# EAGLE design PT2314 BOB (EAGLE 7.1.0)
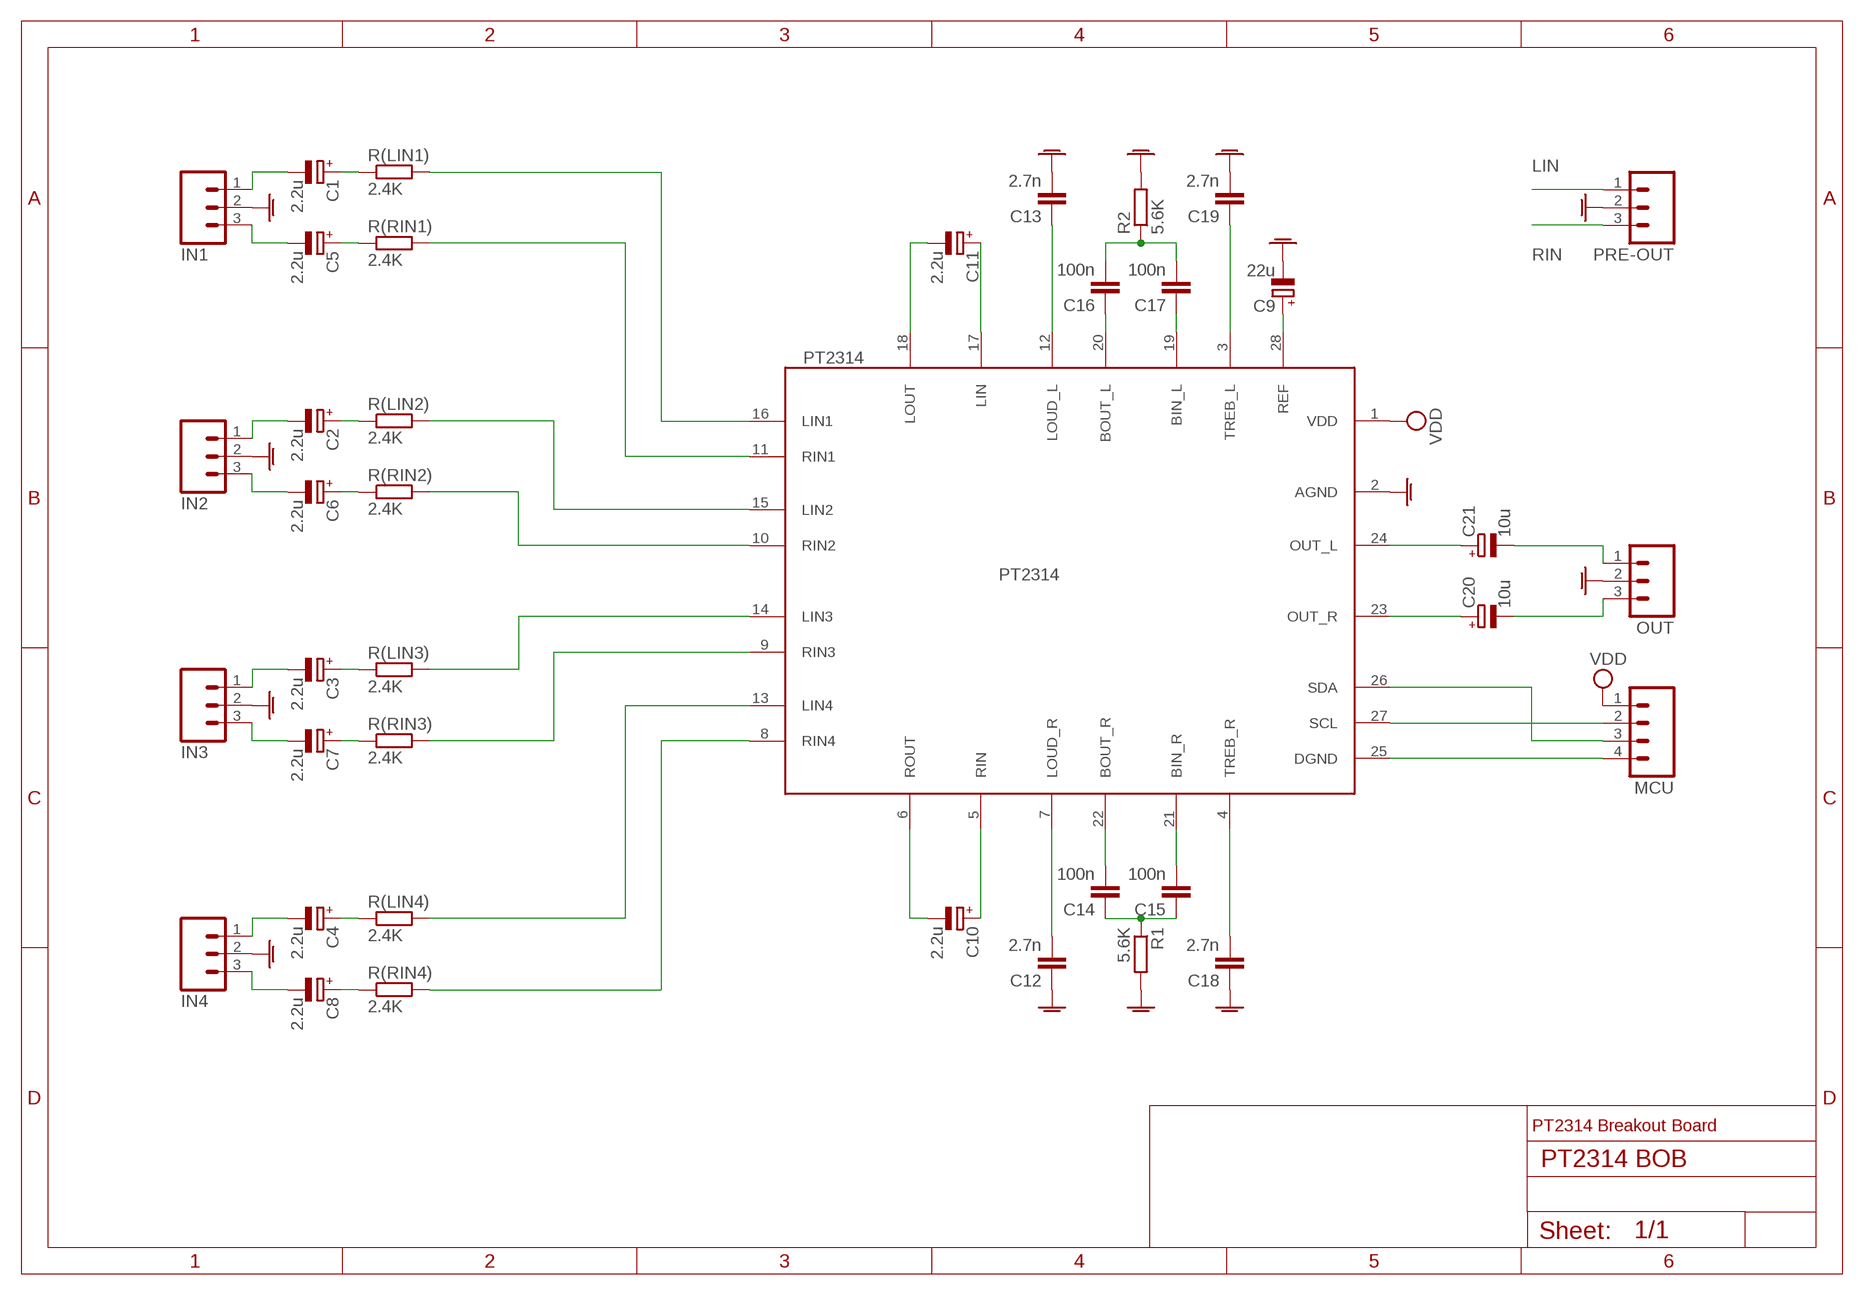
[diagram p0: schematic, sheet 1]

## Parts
C1  2.2u  CPOL-EUSMCZ  [SMC_Z]
C2  2.2u  CPOL-EUSMCZ  [SMC_Z]
C3  2.2u  CPOL-EUSMCZ  [SMC_Z]
C4  2.2u  CPOL-EUSMCZ  [SMC_Z]
C5  2.2u  CPOL-EUSMCZ  [SMC_Z]
C6  2.2u  CPOL-EUSMCZ  [SMC_Z]
C7  2.2u  CPOL-EUSMCZ  [SMC_Z]
C8  2.2u  CPOL-EUSMCZ  [SMC_Z]
C9  22u  CPOL-EUSMCZ  [SMC_Z]
C10  2.2u  CPOL-EUSMCZ  [SMC_Z]
C11  2.2u  CPOL-EUSMCZ  [SMC_Z]
C12  2.7n  C-EUC0603  [C0603]
C13  2.7n  C-EUC0603  [C0603]
C14  100n  C-EUC0603  [C0603]
C15  100n  C-EUC0603  [C0603]
C16  100n  C-EUC0603  [C0603]
C17  100n  C-EUC0603  [C0603]
C18  2.7n  C-EUC0603  [C0603]
C19  2.7n  C-EUC0603  [C0603]
C20  10u  CPOL-EUSMCZ  [SMC_Z]
C21  10u  CPOL-EUSMCZ  [SMC_Z]
IN1  M03PTH  [1X03]
IN2  M03PTH  [1X03]
IN3  M03PTH  [1X03]
IN4  M03PTH  [1X03]
MCU  M04PTH  [1X04]
OUT  M03PTH  [1X03]
PRE-OUT  M03PTH  [1X03]
PT2314  PT2314  [SO-28W]
R1  5.6K  R-EU_R0603  [R0603]
R2  5.6K  R-EU_R0603  [R0603]
R(LIN1)  2.4K  R-EU_R0603  [R0603]
R(LIN2)  2.4K  R-EU_R0603  [R0603]
R(LIN3)  2.4K  R-EU_R0603  [R0603]
R(LIN4)  2.4K  R-EU_R0603  [R0603]
R(RIN1)  2.4K  R-EU_R0603  [R0603]
R(RIN2)  2.4K  R-EU_R0603  [R0603]
R(RIN3)  2.4K  R-EU_R0603  [R0603]
R(RIN4)  2.4K  R-EU_R0603  [R0603]

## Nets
AGND: C9.- C12.1 C13.2 C18.1 C19.2 IN1.2 IN2.2 IN3.2 IN4.2 OUT.2 PRE-OUT.2 PT2314.2(AGND) R1.2 R2.2
B[IN|OUT]_L: C16.2 C17.2 R2.1
B[IN|OUT]_R: C14.1 C15.1 R1.1
BIN_L: C17.1 PT2314.19(BIN_L)
BIN_R: C15.2 PT2314.21(BIN_R)
BOUT_L: C16.1 PT2314.20(BOUT_L)
BOUT_R: C14.2 PT2314.22(BOUT_R)
C1-IN1_L: C1.- IN1.1
C1-R: C1.+ R(LIN1).1
C2-IN2_L: C2.- IN2.1
C2-R: C2.+ R(LIN2).1
C3-IN3_L: C3.- IN3.1
C3-R: C3.+ R(LIN3).1
C4-IN4_L: C4.- IN4.1
C4-R: C4.+ R(LIN4).1
C5-IN1_R: C5.- IN1.3
C5-R: C5.+ R(RIN1).1
C6-IN2_R: C6.- IN2.3
C6-R: C6.+ R(RIN2).1
C7-IN3_R: C7.- IN3.3
C7-R: C7.+ R(RIN3).1
C8-IN4_R: C8.- IN4.3
C8-R: C8.+ R(RIN4).1
C20-OUT_R: C20.- OUT.3
C21-OUT_L: C21.- OUT.1
DGND: MCU.4 PT2314.25(DGND)
LIN: C11.+ PRE-OUT.1 PT2314.17(LIN)
LIN1: PT2314.16(LIN1) R(LIN1).2
LIN2: PT2314.15(LIN2) R(LIN2).2
LIN3: PT2314.14(LIN3) R(LIN3).2
LIN4: PT2314.13(LIN4) R(LIN4).2
LOUT: C11.- PT2314.18(LOUT)
N$1: C19.1 PT2314.3(TREB_L)
N$2: C13.1 PT2314.12(LOUD_L)
N$3: C18.2 PT2314.4(TREB_R)
N$4: C12.2 PT2314.7(LOUD_R)
OUT_L: C21.+ PT2314.24(OUT_L)
OUT_R: C20.+ PT2314.23(OUT_R)
REF: C9.+ PT2314.28(REF)
RIN: C10.+ PRE-OUT.3 PT2314.5(RIN)
RIN1: PT2314.11(RIN1) R(RIN1).2
RIN2: PT2314.10(RIN2) R(RIN2).2
RIN3: PT2314.9(RIN3) R(RIN3).2
RIN4: PT2314.8(RIN4) R(RIN4).2
ROUT: C10.- PT2314.6(ROUT)
SCL: MCU.2 PT2314.27(SCL)
SDA: MCU.3 PT2314.26(SDA)
VDD: MCU.1 PT2314.1(VDD)

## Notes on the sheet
- PT2314 Breakout Board

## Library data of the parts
C1-C11 C20 C21 = rcl:CPOL-EU: POLARIZED CAPACITOR, European symbol
C12-C19 = rcl:C-EU: CAPACITOR, European symbol
IN1-IN4 OUT PRE-OUT = SparkFun-Connectors:M03: Header 3 Standard 3-pin 0.1" header. Use with straight break away headers (SKU : PRT-00116), right angle break away headers (PRT-00553), swiss pins (PRT-00743), machine pins (PRT-00117), and female headers (PRT-00115). Molex polarized connector foot print use with SKU : PRT-08232 with associated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
MCU = SparkFun-Connectors:M04: Header 4 Standard 4-pin 0.1" header. Use with straight break away headers (SKU : PRT-00116), right angle break away headers (PRT-00553), swiss pins (PRT-00743), machine pins (PRT-00117), and female headers (PRT-00115). Molex polarized connector foot print use with SKU : PRT-08231 with associated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
PT2314 = audio-mixer-processor:PT2314: 4-Channel Input Audio Processor
R1 R2 R(LIN1) R(LIN2) R(LIN3) R(LIN4) R(RIN1) R(RIN2) R(RIN3) R(RIN4) = rcl:R-EU_: RESISTOR, European symbol

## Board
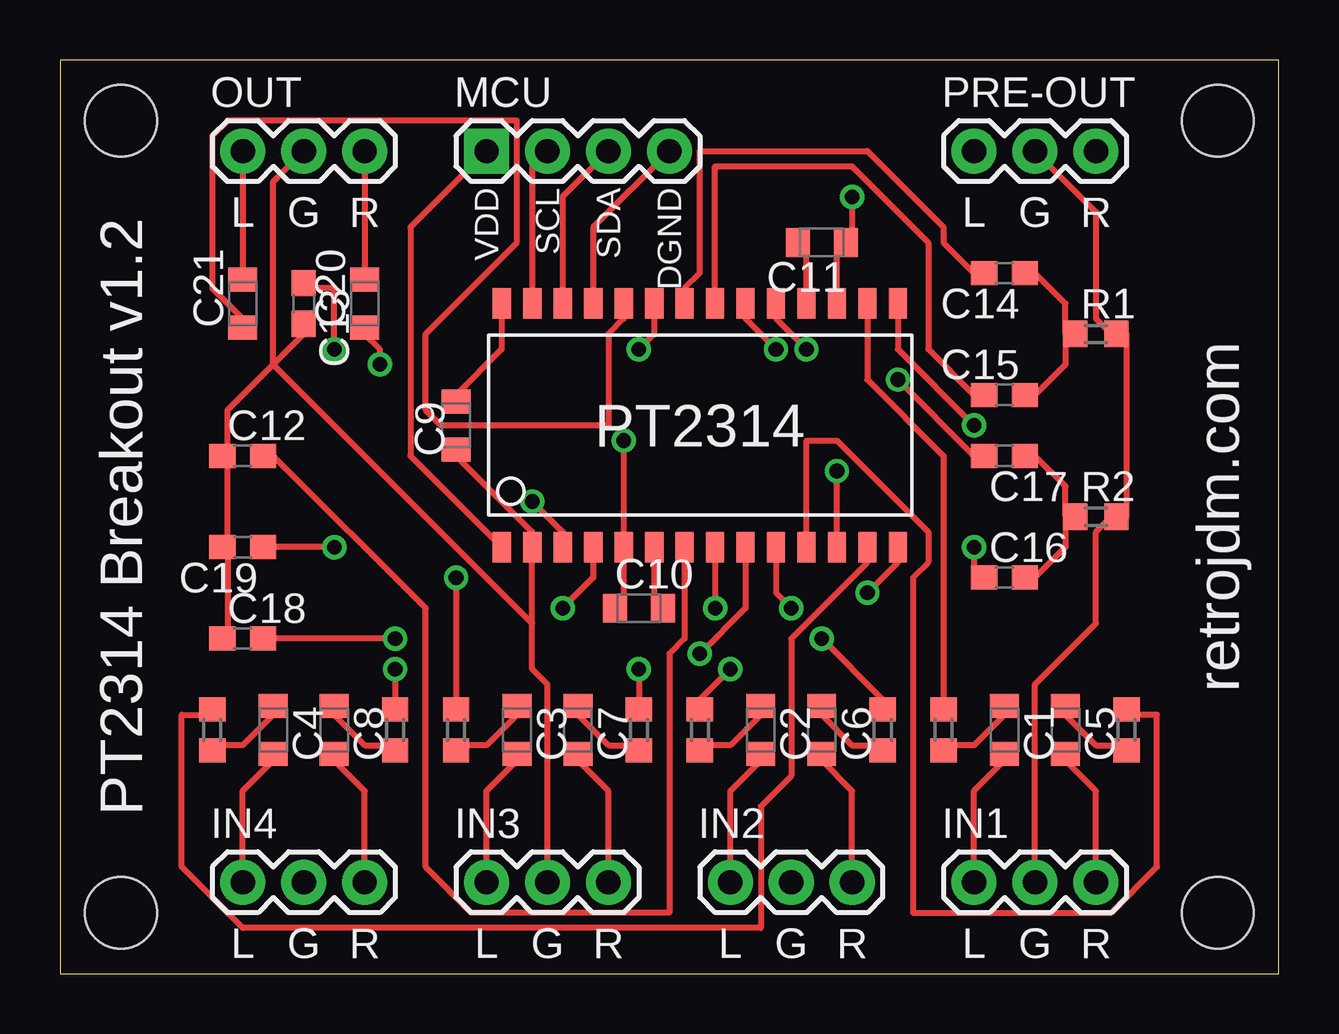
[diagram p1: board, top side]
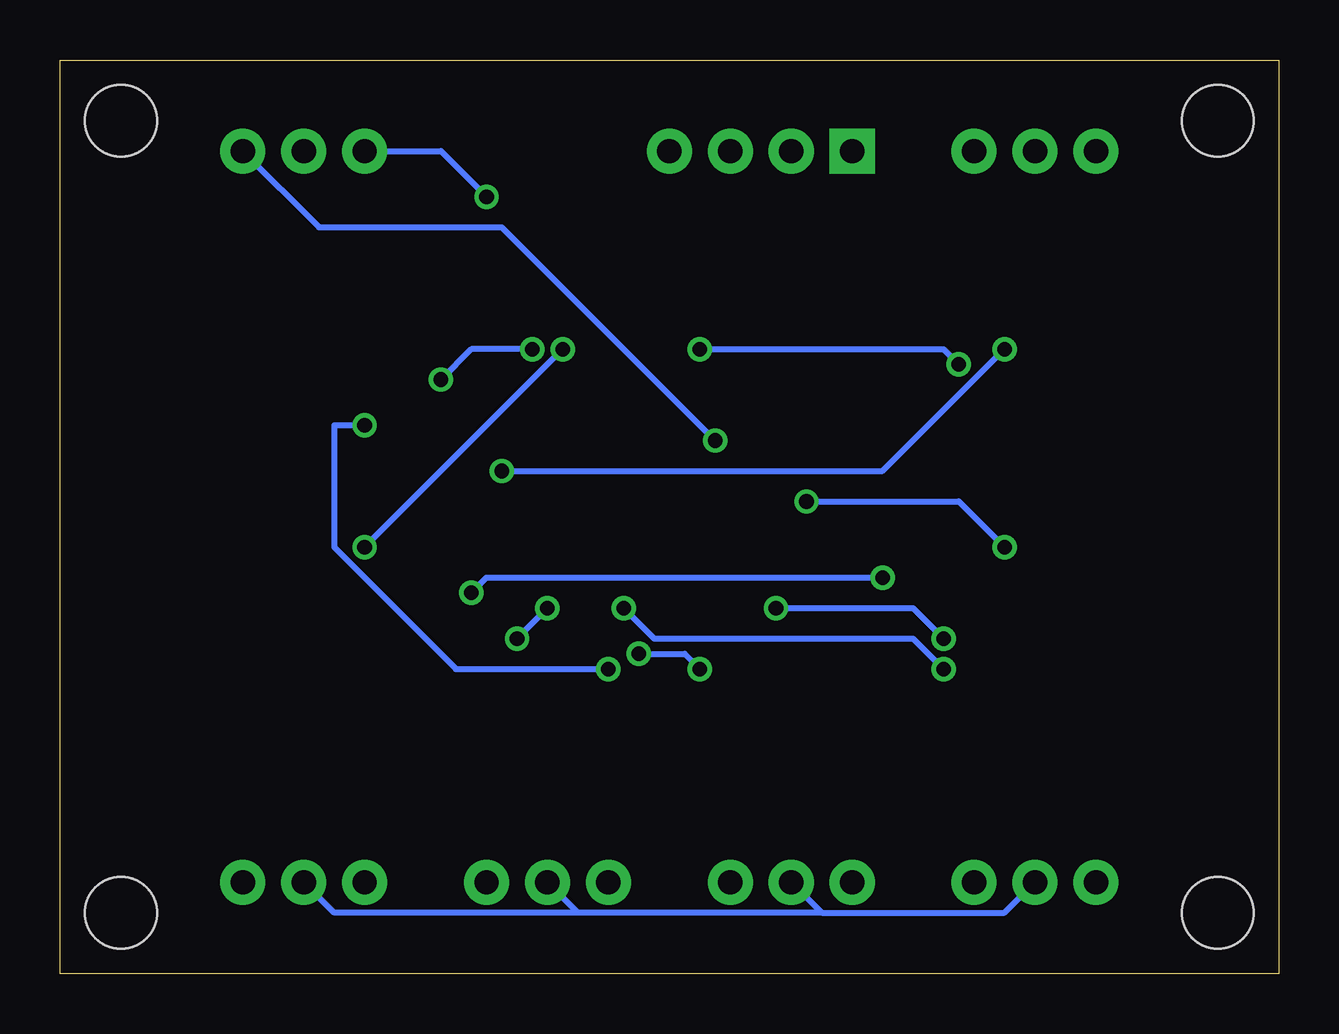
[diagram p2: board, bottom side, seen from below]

Size 50.8 x 38.09 mm. Coordinates in mm from the lower left corner, seen from the top.
Outline: 0,0 50.8,0 50.8,38.09 0,38.09 0,0
Copper layers (1*16): Top 0.035mm / dielectric 1.5mm / Bottom 0.035mm
Design rules "default": minimum track width 10mil, minimum drill 24mil, track to track 8mil, track to pad 8mil, pad to pad 8mil, via to via 8mil, smd to smd 8mil, copper to edge 40mil, drill to drill 8mil, minimum pad ring 10mil, minimum via ring 8mil, stop-mask expansion 4mil, vias tented up to drill 0mil, thermal gap 10mil
Holes 3 mm at 2.54,35.56 2.54,2.54 48.26,2.54 48.26,35.56

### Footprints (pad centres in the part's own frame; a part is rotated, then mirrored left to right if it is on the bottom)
SMC_Z = smd 1 x 1.2: + -1,0; - 1,0
C0603 = smd 1.1 x 1: 1 -0.85,0; 2 0.85,0
1X03 = drill 1.016 pad 1.88: 1 0,0; 2 2.54,0; 3 5.08,0
1X04 = drill 1.016 pad 1.88 square: 1 0,0 | drill 1.016 pad 1.88: 2 2.54,0; 3 5.08,0; 4 7.62,0
SO-28W = smd 0.762 x 1.27: 1 -8.255,-5.08; 2 -6.985,-5.08; 3 -5.715,-5.08; 4 -4.445,-5.08; 5 -3.175,-5.08; 6 -1.905,-5.08; 7 -0.635,-5.08; 8 0.635,-5.08; 9 1.905,-5.08; 10 3.175,-5.08; 11 4.445,-5.08; 12 5.715,-5.08; 13 6.985,-5.08; 14 8.255,-5.08; 15 8.255,5.08; 16 6.985,5.08; 17 5.715,5.08; 18 4.445,5.08; 19 3.175,5.08; 20 1.905,5.08; 21 0.635,5.08; 22 -0.635,5.08; 23 -1.905,5.08; 24 -3.175,5.08; 25 -4.445,5.08; 26 -5.715,5.08; 27 -6.985,5.08; 28 -8.255,5.08
R0603 = smd 1 x 1.1: 1 -0.85,0; 2 0.85,0

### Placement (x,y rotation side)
C1  39.37,10.16 270 top
C2  29.21,10.16 270 top
C3  19.05,10.16 270 top
C4  8.89,10.16 270 top
C5  41.91,10.16 270 top
C6  31.75,10.16 270 top
C7  21.59,10.16 270 top
C8  11.43,10.16 270 top
C9  16.51,22.86 270 top
C10  24.13,15.24 0 top
C11  31.75,30.48 180 top
C12  7.62,21.59 0 top
C13  10.16,27.94 270 top
C14  39.37,29.21 180 top
C15  39.37,24.13 180 top
C16  39.37,16.51 0 top
C17  39.37,21.59 0 top
C18  7.62,13.97 0 top
C19  7.62,17.78 180 top
C20  12.7,27.94 90 top
C21  7.62,27.94 90 top
IN1  38.1,3.81 0 top
IN2  27.94,3.81 0 top
IN3  17.78,3.81 0 top
IN4  7.62,3.81 0 top
MCU  17.78,34.29 0 top
OUT  7.62,34.29 0 top
PRE-OUT  38.1,34.29 0 top
PT2314  26.67,22.86 0 top
R1  43.18,26.67 0 top
R2  43.18,19.05 0 top
R(LIN1)  36.83,10.16 90 top
R(LIN2)  26.67,10.16 90 top
R(LIN3)  16.51,10.16 90 top
R(LIN4)  6.35,10.16 90 top
R(RIN1)  44.45,10.16 90 top
R(RIN2)  34.29,10.16 90 top
R(RIN3)  24.13,10.16 90 top
R(RIN4)  13.97,10.16 90 top

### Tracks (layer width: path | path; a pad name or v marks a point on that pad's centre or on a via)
AGND
  Top 0.254: 6.99,17.78 6.99,13.97 C18.1 | 6.99,17.78 6.99,21.59 | 6.99,17.78 C19.2 | 8.89,25.4 6.99,23.5 6.99,21.59 | 8.89,25.4 10.16,26.67 C13.2 | 6.99,21.59 C12.1 | OUT.2 8.89,33.02 8.89,25.4 | PRE-OUT.2 43.18,31.75 43.18,27.3 43.81,26.67 R1.2 44.45,26.67 44.45,19.05 R2.2 43.81,19.05 43.18,18.41 43.18,14.61 40.64,12.06 IN1.2 | C9.- 16.51,21.59 19.68,18.41 PT2314.2 19.68,14.61 | 19.68,14.61 19.68,12.7 20.32,12.06 IN3.2 | 19.68,14.61 8.89,25.4
  Bottom 0.254: IN4.2 11.43,2.54 19.05,2.54 | IN3.2 19.05,2.54 | 29.21,2.54 IN2.2 | 19.05,2.54 29.21,2.54 | IN1.2 39.37,2.54 29.21,2.54
B[IN|OUT]_L
  Top 0.254: 41.91,19.05 41.91,17.78 40.64,16.51 C16.2 | 41.91,19.05 41.91,20.32 40.64,21.59 C17.2 | 41.91,19.05 R2.1
B[IN|OUT]_R
  Top 0.254: 41.91,26.67 41.91,25.4 40.64,24.13 C15.1 | 41.91,26.67 41.91,27.94 40.64,29.21 C14.1 | 41.91,26.67 R1.1
BIN_L  (via drill 0.61)
  Top 0.254: v34.92,24.77 38.1,21.59 C17.1 | v31.11,26.04 29.84,27.3 PT2314.19
  Bottom 0.254: v34.92,24.77 33.66,26.04 v31.11,26.04
BIN_R
  Top 0.254: PT2314.21 27.3,33.66 33.02,33.66 36.2,30.48 36.2,26.04 38.1,24.13 C15.2
BOUT_L  (via drill 0.61)
  Top 0.254: v38.1,17.78 38.1,16.51 C16.1 | v29.84,26.04 28.57,27.3 PT2314.20
  Bottom 0.254: v29.84,26.04 v38.1,17.78
BOUT_R
  Top 0.254: PT2314.22 26.04,28.57 26.67,29.21 26.67,34.29 33.66,34.29 36.83,31.11 36.83,30.48 38.1,29.21 C14.2
C1-IN1_L
  Top 0.254: IN1.1 38.1,7.62 39.37,8.89 C1.-
C1-R
  Top 0.254: R(LIN1).1 36.83,9.53 38.1,9.53 39.37,10.79 C1.+
C2-IN2_L
  Top 0.254: IN2.1 27.94,7.62 29.21,8.89 C2.-
C2-R
  Top 0.254: R(LIN2).1 26.67,9.53 27.94,9.53 29.21,10.79 C2.+
C3-IN3_L
  Top 0.254: IN3.1 17.78,7.62 19.05,8.89 C3.-
C3-R
  Top 0.254: R(LIN3).1 16.51,9.53 17.78,9.53 19.05,10.79 C3.+
C4-IN4_L
  Top 0.254: IN4.1 7.62,7.62 8.89,8.89 C4.-
C4-R
  Top 0.254: R(LIN4).1 6.35,9.53 7.62,9.53 8.89,10.79 C4.+
C5-IN1_R
  Top 0.254: IN1.3 43.18,7.62 41.91,8.89 C5.-
C5-R
  Top 0.254: R(RIN1).1 44.45,9.53 43.18,9.53 41.91,10.79 C5.+
C6-IN2_R
  Top 0.254: IN2.3 33.02,7.62 31.75,8.89 C6.-
C6-R
  Top 0.254: R(RIN2).1 34.29,9.53 33.02,9.53 31.75,10.79 C6.+
C7-IN3_R
  Top 0.254: IN3.3 22.86,7.62 21.59,8.89 C7.-
C7-R
  Top 0.254: R(RIN3).1 24.13,9.53 22.86,9.53 21.59,10.79 C7.+
C8-IN4_R
  Top 0.254: IN4.3 12.7,7.62 11.43,8.89 C8.-
C8-R
  Top 0.254: R(RIN4).1 13.97,9.53 12.7,9.53 11.43,10.79 C8.+
C20-OUT_R
  Top 0.254: OUT.3 C20.-
C21-OUT_L
  Top 0.254: OUT.1 C21.-
DGND
  Top 0.254: PT2314.25 22.23,31.11 MCU.4
LIN  (via drill 0.61)
  Top 0.254: PT2314.17 32.38,30.48 C11.+ 33.02,30.48 v33.02,32.38
  Bottom 0.254: v33.02,32.38 34.92,34.29 PRE-OUT.1
LIN1
  Top 0.254: R(LIN1).2 36.83,21.59 33.66,24.77 PT2314.16
LIN2  (via drill 0.61)
  Top 0.254: v27.94,12.7 26.67,11.43 R(LIN2).2 | v38.1,22.86 34.92,26.04 PT2314.15
  Bottom 0.254: v27.94,12.7 34.29,12.7 39.37,17.78 39.37,22.86 v38.1,22.86
LIN3  (via drill 0.61)
  Top 0.254: v16.51,16.51 R(LIN3).2 | v33.66,15.88 34.92,17.14 PT2314.14
  Bottom 0.254: v16.51,16.51 33.02,16.51 v33.66,15.88
LIN4
  Top 0.254: PT2314.13 33.66,17.14 30.48,13.97 30.48,8.26 29.21,6.99 29.21,1.91 7.62,1.91 5.08,4.45 5.08,10.79 6.35,10.79 R(LIN4).2
LOUT
  Top 0.254: PT2314.18 31.11,30.48 C11.-
N$1  (via drill 0.61)
  Top 0.254: v11.43,17.78 C19.1 | v19.68,19.68 20.95,18.41 PT2314.3
  Bottom 0.254: v11.43,17.78 13.34,19.68 v19.68,19.68
N$2  (via drill 0.61)
  Top 0.254: v11.43,26.04 11.43,28.57 10.16,28.57 C13.1 | PT2314.12 v32.38,20.95
  Bottom 0.254: v11.43,26.04 16.51,20.95 v32.38,20.95
N$3  (via drill 0.61)
  Top 0.254: v13.97,13.97 C18.2 | v20.95,15.24 22.23,16.51 PT2314.4
  Bottom 0.254: v13.97,13.97 15.24,15.24 v20.95,15.24
N$4
  Top 0.254: PT2314.7 26.04,13.97 25.4,13.34 25.4,2.54 17.14,2.54 15.24,4.45 15.24,15.24 8.89,21.59 C12.2
OUT_L
  Top 0.254: PT2314.24 23.5,27.3 22.86,26.67 22.86,22.86 15.88,22.86 15.24,23.5 15.24,26.67 19.05,30.48 19.05,35.56 6.99,35.56 6.35,34.92 6.35,28.57 7.62,27.3 C21.+
OUT_R  (via drill 0.61)
  Top 0.254: v13.34,25.4 13.34,26.04 12.7,26.67 C20.+ | v24.13,26.04 24.77,26.67 PT2314.23
  Bottom 0.254: v13.34,25.4 13.97,26.04 v24.13,26.04
REF
  Top 0.254: PT2314.28 18.41,26.04 16.51,24.13 C9.+
RIN  (via drill 0.61)
  Top 0.254: C10.+ 23.5,15.24 PT2314.5 v23.5,22.23
  Bottom 0.254: v23.5,22.23 32.38,31.11 40.01,31.11 PRE-OUT.3
RIN1
  Top 0.254: PT2314.11 31.11,22.23 32.38,22.23 36.2,18.41 36.2,17.14 35.56,16.51 35.56,2.54 43.81,2.54 45.72,4.45 45.72,10.79 44.45,10.79 R(RIN1).2
RIN2  (via drill 0.61)
  Top 0.254: v31.75,13.97 34.29,11.43 R(RIN2).2 | v30.48,15.24 29.84,15.88 PT2314.10
  Bottom 0.254: v30.48,15.24 v31.75,13.97
RIN3  (via drill 0.61)
  Top 0.254: v24.13,12.7 R(RIN3).2 | v26.67,13.34 28.57,15.24 PT2314.9
  Bottom 0.254: v24.13,12.7 24.77,13.34 v26.67,13.34
RIN4  (via drill 0.61)
  Top 0.254: v13.97,12.7 R(RIN4).2 | PT2314.8 v27.3,15.24
  Bottom 0.254: v13.97,12.7 15.24,13.97 26.04,13.97 v27.3,15.24
ROUT
  Top 0.254: PT2314.6 24.77,15.24 C10.-
SCL
  Top 0.254: PT2314.27 19.68,33.66 MCU.2
SDA
  Top 0.254: PT2314.26 20.95,32.38 MCU.3
VDD
  Top 0.254: PT2314.1 14.61,21.59 14.61,31.11 MCU.1

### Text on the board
tNames: VDD | SCL | SDA | DGND | L | G | R | L | G | R | PT2314 Breakout v1.2 | retrojdm.com | L | G | R | L | G | R | L | G | R | L | G | R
